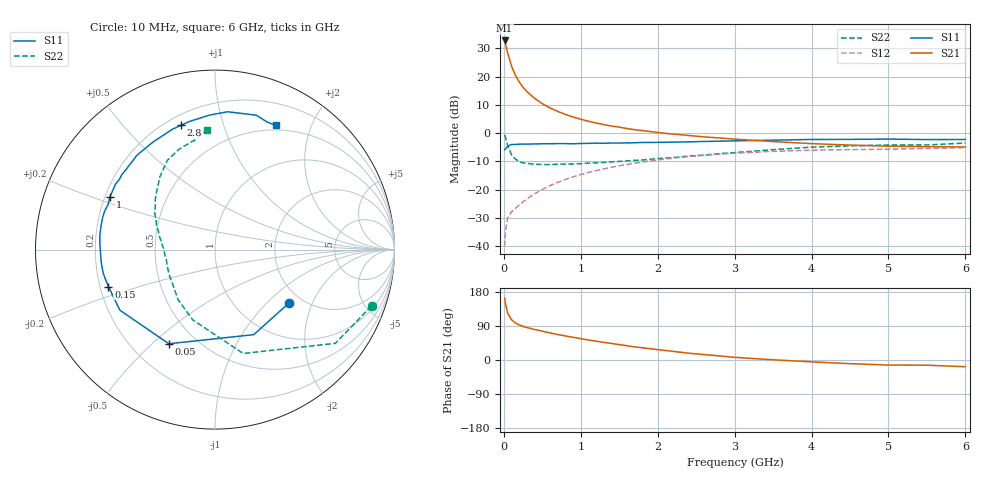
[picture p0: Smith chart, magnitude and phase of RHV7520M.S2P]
! SIEMENS Small Signal Semiconductors
! BFR106
! Si NPN RF Bipolar Junction Transistor in SOT23
! VCE = 0.75 V  IC = 20 mA
! Common Emitter S-Parameters:  August  1996
# GHz  S  MA  R  50
!  f  S11  S21  S12  S22
! GHz  MAG  ANG  MAG  ANG  MAG  ANG  MAG  ANG
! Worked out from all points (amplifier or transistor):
!   36 points, 10 MHz to 6 GHz, reference 50 ohm
!   highest |S21| = 32.8 dB at 10 MHz (marker M1)
!   |S21| within 3 dB of that: start of sweep to 37.81 MHz
!   unconditionally stable (mu >= 1): 318.7 MHz to end of sweep
!   at 250 MHz: K = 0.92, MSG = 20.3 dB, |S12| = -24.4 dB
!   at 1.4 GHz: K = 1.10, MAG = 5.4 dB, |S12| = -12.1 dB
!   at 6 GHz: K = 1.03, MAG = -0.9 dB, |S12| = -5.2 dB
!   S11 on the Smith chart (normalised r, x): 10 MHz: 1.71, -1.37; 50 MHz: 0.36, -0.57; 150 MHz: 0.23, -0.16; 1 GHz: 0.22, +0.22; 2.8 GHz: 0.26, +0.73; 6 GHz: 0.44, +1.51
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0.01  0.5087 -35.7  43.88 163.3  0.0099 77.7  0.927 -19.8
0.02  0.5207 -65.5  39.61 149.8  0.0176 66.4  0.85 -37.9
0.05  0.5842 -116.1  26.31 123.8  0.0312 48.9  0.5998 -74.8
0.1  0.6284 -147.5  15.4 106.1  0.0405 44.7  0.4103 -107.7
0.15  0.6285 -160.8  10.59 97.7  0.0463 47.2  0.3469 -126.4
0.2  0.6365 -167.8  8.084 92.6  0.0534 50.5  0.3112 -137.5
0.25  0.6379 -173.2  6.471 88.6  0.0605 53.0  0.2962 -146.6
0.3  0.6376 -177.1  5.431 85.7  0.0681 55.9  0.2901 -152.2
0.4  0.6427 176.8  4.123 80.6  0.0838 59.2  0.2814 -160.8
0.5  0.6467 172.7  3.323 76.0  0.1002 60.8  0.2775 -166.6
0.6  0.6484 168.0  2.794 71.5  0.1171 61.2  0.2769 -170.4
0.7  0.6514 164.0  2.425 67.2  0.1339 61.0  0.2805 -173.8
0.8  0.6511 160.8  2.144 63.6  0.1508 60.4  0.2828 -177.2
1  0.6546 153.5  1.76 56.4  0.1842 58.7  0.2876 178.1
1.1  0.6579 150.3  1.624 52.9  0.2005 57.5  0.2939 176.0
1.6  0.6702 135.3  1.201 37.6  0.2781 50.1  0.3219 165.5
2.2  0.6921 119.8  0.959 22.8  0.3591 40.0  0.3684 153.1
2.8  0.7183 105.2  0.82 10.8  0.4217 29.9  0.4321 140.5
3.5  0.7501 92.3  0.707 0.5  0.4752 18.8  0.5085 127.2
4.5  0.7739 78.2  0.613 -9.7  0.5094 4.8  0.5941 109.7
5.5  0.7681 67.9  0.575 -13.7  0.5352 -3.5  0.6171 101.2
6  0.7704 63.9  0.567 -17.8  0.5515 -9.8  0.6658 94.0
